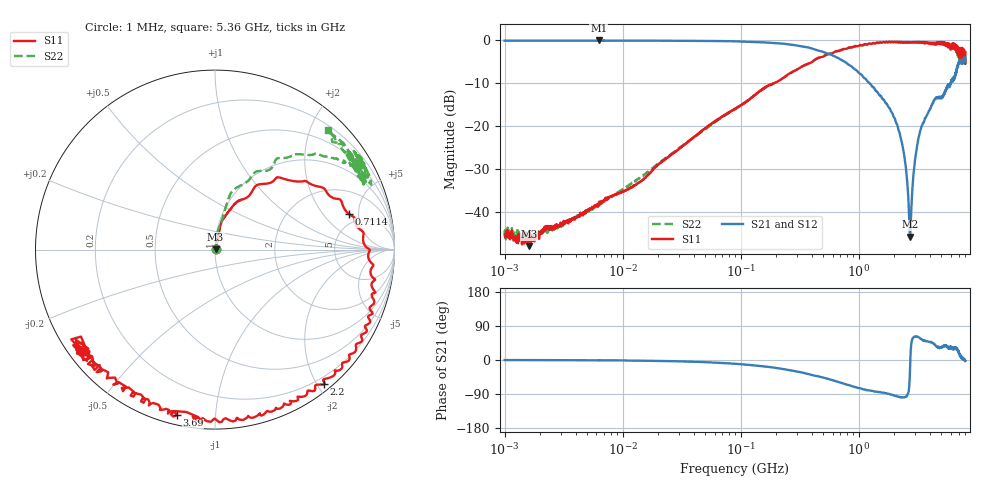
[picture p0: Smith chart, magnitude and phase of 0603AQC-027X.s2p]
!s-Parameter Generated by FASTRON Sdn. Bhd.
!FASTRON P/N : 0603AQC-027X
!Keysight Technologies: E5071C_MY46733604_B.14.02
!Date: Thu Jun 25 13:52:56 2026
!Version  :Rev00  Thu Jun 25 13:52:56 2026
!Data & Calibration Information:
!Freq  S11:SOLT2(ON)  S21:SOLT2(ON)  S12:SOLT2(ON)  S22:SOLT2(ON)
!PortZ  Port1:50+j0  Port2:50+j0
!When reading reference impedance value at option line is always used.
! Remarks : This data is being provided solely for informational purposes.
# Hz S dB R 50
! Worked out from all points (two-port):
!   1601 points, 1 MHz to 8 GHz, reference 50 ohm
!   highest |S21| = -0.01 dB at 6.268 MHz (marker M1); lowest = -45.8 dB at 2.722 GHz (marker M2)
!   |S21| within 3 dB of the highest: start of sweep to 536.8 MHz
!   lowest |S11| = -48.0 dB at 1.605 MHz (marker M3), VSWR 1.01, Z = 50.4 + j0.18 ohm
!   |S11| at or under -10 dB: start of sweep to 189.8 MHz
!   |S22| runs from -47.3 to -0.3 dB; largest |S21 - S12| = 0.019
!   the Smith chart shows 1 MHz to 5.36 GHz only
!   S11 on the Smith chart (normalised r, x): 1 MHz: 1.01, +0.00; 711.4 MHz: 3.91, +3.83; 2.2 GHz: 0.09, -2.09; 3.69 GHz: 0.04, -0.79; 5.36 GHz: 0.04, -0.33
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1000000  -45.30 13.1  -0.05 -0.2  -0.05 -0.1  -44.90 15.3
1604653  -48.00 26.7  -0.04 -0.3  -0.05 -0.1  -45.70 14.4
4479405  -40.50 57.4  -0.05 -0.5  -0.06 -0.6  -40.50 64.2
6268472  -38.00 58.7  -0.01 -1.2  -0.10 -0.2  -38.90 65.8
2.00676e7  -29.00 74.2  -0.07 -2.4  -0.07 -2.3  -28.70 81.0
8.994653e7  -15.90 76.6  -0.21 -10.0  -0.21 -10.0  -16.00 76.9
2.100621e8  -9.44 58.8  -0.66 -22.0  -0.67 -22.0  -9.42 73.6
4.006501e8  -5.06 44.2  -1.86 -39.5  -1.86 -39.5  -4.95 55.3
7.113666e8  -2.24 14.8  -4.55 -60.3  -4.55 -60.4  -2.19 43.6
1.171668e9  -0.98 -12.2  -9.35 -79.7  -9.35 -79.8  -0.90 30.5
1.7949e9  -0.35 -35.1  -15.60 -89.0  -15.70 -89.2  -0.37 32.7
2.199693e9  -0.31 -51.0  -21.30 -96.9  -21.30 -96.9  -0.42 30.7
2.44288e9  -0.54 -60.7  -27.40 -98.9  -27.50 -99.2  -0.46 28.6
2.721653e9  -0.46 -69.0  -45.80 -15.8  -45.80 -17.2  -0.48 33.6
3.061592e9  -0.42 -79.2  -26.00 62.5  -26.00 62.4  -0.46 34.2
3.689925e9  -0.47 -103.0  -18.00 49.9  -18.00 49.7  -0.56 29.2
4.744521e9  -0.42 -138.0  -13.50 32.8  -13.50 32.6  -0.71 24.2
5.360342e9  -0.61 -143.0  -12.30 39.0  -12.30 38.7  -0.72 46.6
6.110812e9  -1.26 -168.0  -9.40 29.1  -9.39 28.7  -1.64 36.0
6.766244e9  -2.85 -166.0  -6.35 31.0  -6.32 30.4  -2.88 64.7
7.383122e9  -2.73 150.0  -5.04 4.8  -5.06 4.0  -3.53 41.5
8e9  -2.78 145.0  -4.37 -2.6  -4.40 -3.3  -4.22 53.5
